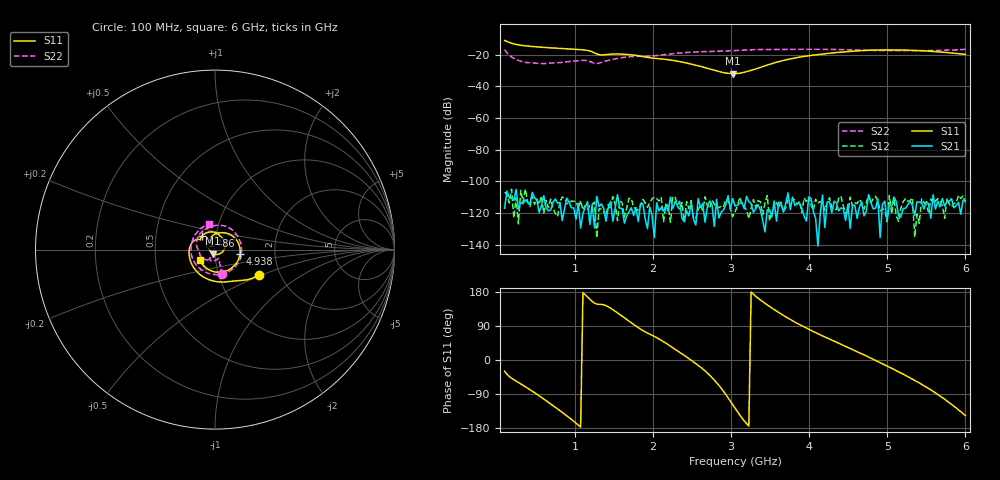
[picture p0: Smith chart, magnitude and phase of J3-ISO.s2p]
!Agilent Technologies,E8364B,MY43040379,A.07.50.67
!Agilent E8364B: A.07.50.67
!Date: Tuesday, March 24, 2026 11:06:47
!Correction: S11(Full 2 Port(1,2))
!S21(Full 2 Port(1,2))
!S12(Full 2 Port(1,2))
!S22(Full 2 Port(1,2))
!S2P File: Measurements: S11, S21, S12, S22:
# Hz S  dB  R 50
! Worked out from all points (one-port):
!   201 points, 100 MHz to 6 GHz, reference 50 ohm
!   lowest |S11| = -32.0 dB at 3.021 GHz (marker M1), VSWR 1.05, Z = 48.8 - j2.18 ohm
!   |S11| at or under -10 dB: start of sweep to end of sweep
!   S11 on the Smith chart (normalised r, x): 100 MHz: 1.56, -0.48; 1.486 GHz: 0.86, +0.13; 4.938 GHz: 1.32, -0.07; 6 GHz: 0.84, -0.10
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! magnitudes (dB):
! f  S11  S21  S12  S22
! 100 MHz  -11.0  -117.0  -106.8  -16.8
! 159 MHz  -12.2  -110.2  -113.7  -20.2
! 218 MHz  -13.2  -112.1  -123.1  -22.3
! 395 MHz  -14.5  -113.1  -112.9  -25.0
! 601.5 MHz  -15.4  -109.1  -120.1  -25.6
! 1.103 GHz  -16.9  -120.2  -118.1  -23.5
! 1.28 GHz  -19.5  -109.5  -135.6  -25.6
! 1.486 GHz  -19.6  -125.2  -109.6  -22.9
! 1.722 GHz  -20.1  -116.7  -110.8  -21.3
! 2.076 GHz  -22.5  -118.7  -112.5  -20.4
! 2.401 GHz  -24.9  -125.5  -125.5  -18.7
! 2.902 GHz  -31.3  -118.1  -116.2  -17.7
! 3.021 GHz  -32.0  -110.9  -122.4  -17.4
! 3.05 GHz  -31.9  -115.5  -119.1  -17.3
! 3.227 GHz  -30.3  -112.8  -123.6  -16.9
! 3.699 GHz  -23.3  -114.0  -116.8  -16.6
! 4.053 GHz  -20.2  -119.0  -118.5  -16.5
! 4.525 GHz  -17.9  -129.8  -110.0  -16.9
! 4.938 GHz  -17.0  -114.5  -117.3  -17.3
! 5.027 GHz  -17.0  -115.0  -108.9  -17.4
! 5.498 GHz  -17.6  -112.7  -114.6  -17.4
! 6 GHz  -19.8  -112.0  -113.4  -16.6
